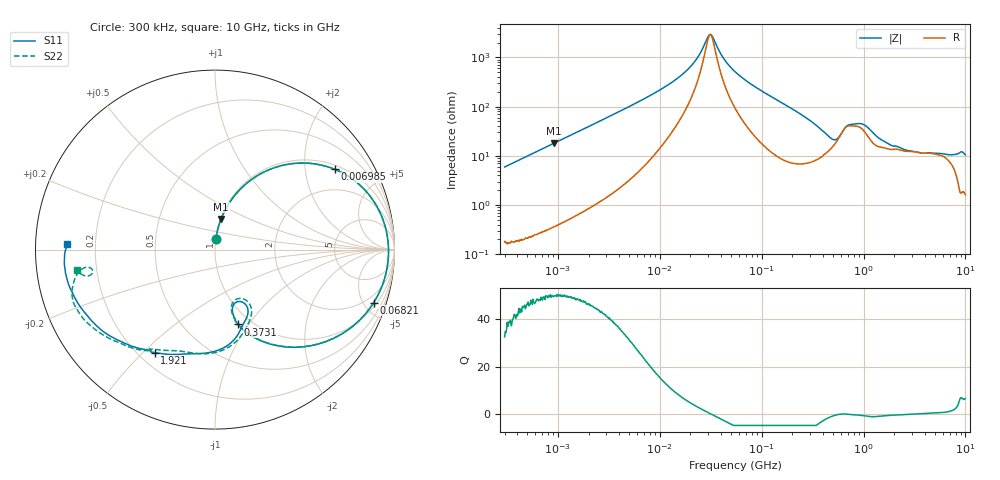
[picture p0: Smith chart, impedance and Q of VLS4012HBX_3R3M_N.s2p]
! S-Parameter Data Generated by TDK Corporation
! Copyright(C) 2023 TDK Corporation.
! All Rights Reserved.
! TDK P/N: VLS4012HBX-3R3M-N (Inductor)
! Property: L=3.3uH at 1MHz
! Size(LxWxT): 4x4x1.2mm
! Model Type: s2p (Touchstone File Format Version 1.0)
! Frequency: DC=Yes Start=0.3MHz Stop=10000MHz 802points Log-sweep
! Model Generated on June 16, 2023
! Port Assignments:
!  1 ---@@@--- 2
! Applicable Conditions:
!  Temperature = 25 degC
!  DC Bias Current = 0 A
!  Small Signal Operation
! Terms and conditions regarding TDK Simulation Models
! (1)This simulation model is being provided solely for informational purposes. Please refer to the specifications of the products in terms of detailed characteristics of such products.
! (2)In no event shall TDK Corporation of any of its subsidiaries be liable for any loss or damage arising, directly or indirectly,
!  From any information contained in this simulation model, including, but not limited to loss or damages arising from any inaccuracies, omissions or errors in connection with such information.
! (3)Any and all copyrights on this simulation model are owned by TDK Corporation.
!  Duplication or redistribution of this simulation model without prior written permission from TDK Corporation is prohibited.
! (4)This simulation model is subject to any modification or change without any prior notice.
! (5)Neither TDK Corporation nor any of its subsidiaries shall make any warranty, express or implied,
!  Including but not limited to the correctness, implied warranties of merchantability and fitness for a particular purpose with respect to this simulation models.
! (6)The use of this simulation model shall be deemed to have consented to the terms and conditions hereof.
# Hz S MA R 50
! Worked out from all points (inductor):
!   801 points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, 300 kHz to 10 GHz, reference 50 ohm
!   read as one part in series: L = 3.14 uH near 318.3 kHz
!   highest Q = 50.1 at 905.9 kHz (marker M1), where L = 3.13 uH
!   self-resonance near 31.37 MHz
!   S11 on the Smith chart (normalised r, x): 300 kHz: 1.00, +0.12; 6.985 MHz: 1.14, +2.88; 68.21 MHz: 1.30, -5.87; 373.1 MHz: 0.87, -0.89; 1.921 GHz: 0.26, -0.54; 10 GHz: 0.10, +0.02
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300000  0.05878 84.8  0.9964 -3.4  0.9965 -3.4  0.05857 84.8
905948  0.1746 78.7  0.9812 -10.1  0.981 -10.1  0.1745 78.7
1713600  0.3164 70.3  0.942 -18.5  0.942 -18.5  0.3165 70.3
4001173  0.6122 50.5  0.7741 -37.9  0.774 -37.9  0.6121 50.5
6985119  0.8035 33.8  0.562 -53.7  0.5621 -53.7  0.8034 33.8
9671944  0.8803 24.5  0.4227 -62.0  0.4227 -62.0  0.8803 24.5
1.945436e7  0.9565 7.9  0.1572 -70.5  0.1572 -70.5  0.9566 7.9
3.118733e7  0.9669 -1.5  0.03304 -4.5  0.03304 -4.5  0.9671 -1.4
5.477226e7  0.9501 -13.2  0.184 66.5  0.184 66.5  0.9504 -13.1
6.820897e7  0.9323 -18.5  0.2618 64.3  0.2618 64.3  0.9326 -18.4
1.585658e8  0.7595 -44.8  0.6009 41.5  0.601 41.5  0.7596 -44.6
3.126428e8  0.5052 -68.4  0.8028 14.7  0.8028 14.7  0.5047 -68.3
3.730642e8  0.4366 -72.9  0.8257 7.1  0.8258 7.1  0.4351 -73.0
5.745924e8  0.3169 -66.0  0.7748 -13.5  0.7749 -13.5  0.3013 -65.8
7.956093e8  0.4424 -69.0  0.6423 -17.5  0.6424 -17.5  0.4573 -66.6
1.10164e9  0.5602 -88.0  0.6416 -19.0  0.6417 -19.0  0.574 -90.2
1.767019e9  0.6465 -115.9  0.6277 -39.1  0.6278 -39.1  0.6339 -117.9
1.920785e9  0.6647 -120.4  0.6066 -43.3  0.6067 -43.3  0.6538 -121.9
4.34106e9  0.8074 -154.5  0.3737 -77.2  0.3737 -77.3  0.8136 -148.8
6.899057e9  0.8412 -169.2  0.2735 -96.0  0.2736 -96.1  0.8369 -161.9
8.322921e9  0.8393 -177.3  0.2346 -107.1  0.2347 -107.2  0.7444 -171.8
1e10  0.8257 178.0  0.2221 -111.8  0.2222 -111.8  0.7755 -171.5
